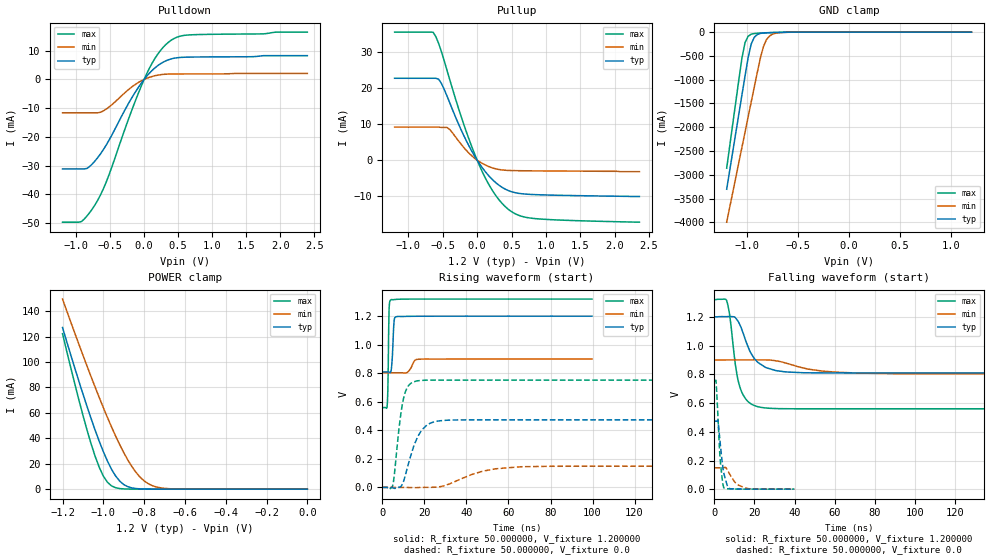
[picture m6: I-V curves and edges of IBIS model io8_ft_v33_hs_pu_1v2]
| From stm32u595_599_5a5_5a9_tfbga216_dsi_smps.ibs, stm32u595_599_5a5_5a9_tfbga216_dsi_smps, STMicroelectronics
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|   Model io8_ft_v33_hs_pu_1v2
[Model]  io8_ft_v33_hs_pu_1v2
Model_type I/O
Polarity   Non-Inverting
Enable   Active-Low
Vinl =   0.360000V
Vinh =   0.840000V
Vmeas =  0.600000V
Cref =   50.000000pF
Rref =   100.000000M
Vref =   0.0V
C_comp   2.887200pF   2.816900pF   2.935200pF
[Temperature Range]   25.000000   0.140000k   -40.000000
[Pullup Reference]   1.200000V   0.900000V   1.320000V
[Pulldown Reference]   0.0V   0.0V   0.0V
[POWER Clamp Reference]   1.200000V   0.900000V   1.320000V
[GND Clamp Reference]   0.0V   0.0V   0.0V
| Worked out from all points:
|   slope of the pulldown table from 0 to 0.18 V, typ, clamps not added: 40.7 ohm
|   slope of the pullup table from 0 to 0.18 V, typ, clamps not added: 39.5 ohm
|   GND clamp passes 1 mA (typ) near -0.51 V on its own axis
|   POWER clamp passes 1 mA (typ) near -0.86 V on its own axis
|   rising waveform, R_fixture 50.000000, V_fixture 1.200000: 20-80 % time 756ps typ, 2.05ns min, 445ps max; typ from 0.809 V to 1.2 V
|   rising waveform, R_fixture 50.000000, V_fixture 0.0: 20-80 % time 6.66ns typ, 16.9ns min, 3.63ns max; typ from 0.001 V to 0.474 V
|   falling waveform, R_fixture 50.000000, V_fixture 1.200000: 20-80 % time 7.98ns typ, 18.6ns min, 4.69ns max; typ from 1.2 V to 0.809 V
|   falling waveform, R_fixture 50.000000, V_fixture 0.0: 20-80 % time 2.51ns typ, 4.77ns min, 1.85ns max; typ from 0.474 V to 0.001 V
[Pulldown]
|Voltage   I(typ)   I(min)   I(max)
-1.2V     -31.16mA   -11.61mA   -49.71mA
-920mV    -31.16mA   -11.61mA   -49.49mA
-840mV    -31mA      -11.61mA   -47.54mA
-720mV    -28.32mA   -11.61mA   -43.58mA
-560mV    -22.95mA   -10.37mA   -35.89mA
-200mV    -7.146mA   -2.964mA   -11.89mA
0V        0A         0A         0A
160mV     4.047mA    1.298mA    7.361mA
360mV     6.869mA    1.87mA     13mA
480mV     7.543mA    1.91mA     14.69mA
640mV     7.765mA    1.923mA    15.46mA
2.4V      8.292mA    2.092mA    16.49mA
[Pullup]
|Voltage   I(typ)   I(min)   I(max)
-1.2V     22.73mA    9.162mA    35.55mA
-640mV    22.73mA    9.162mA    35.51mA
-560mV    22.48mA    9.162mA    32.41mA
-520mV    21.33mA    9.091mA    30.16mA
-400mV    15.99mA    8.534mA    22.45mA
-200mV    7.069mA    3.642mA    10.26mA
40mV      -1.16mA    -508.1uA   -1.774mA
240mV     -5.73mA    -2.256mA   -8.953mA
480mV     -8.639mA   -2.877mA   -14.04mA
640mV     -9.31mA    -2.942mA   -15.55mA
880mV     -9.601mA   -2.986mA   -16.29mA
2.36V     -10.1mA    -3.2mA     -17.23mA
[GND_clamp]
|Voltage   I(typ)   I(min)   I(max)
-1.2V     -3.305A    -3.998A    -2.862A
-1.05V    -1.316A    -2.418A    -539.3mA
-1.02V    -921mA     -2.103A    -218.8mA
-990mV    -539.5mA   -1.788A    -87.43mA
-960mV    -252.1mA   -1.474A    -44.36mA
-930mV    -110.5mA   -1.16A     -30.32mA
-870mV    -28.03mA   -549.1mA   -21.09mA
-840mV    -18.43mA   -305.6mA   -18.27mA
-810mV    -13.9mA    -159.7mA   -15.73mA
-780mV    -11.23mA   -82.35mA   -13.37mA
-600mV    -2.976mA   -4.272mA   -3.058mA
1.2V      0A         14.74nA    0A
[POWER_clamp]
|Voltage   I(typ)   I(min)   I(max)
-1.2V     127mA      149.4mA    122.2mA
-1.12V    84.98mA    114mA      70.29mA
-1.06V    55.52mA    88.42mA    35.69mA
-1.02V    37.64mA    72.04mA    17.19mA
-1V       29.52mA    64.13mA    10.33mA
-960mV    15.7mA     48.99mA    2.597mA
-900mV    3.636mA    28.77mA    209uA
-840mV    503.6uA    13.24mA    43.76uA
-800mV    129.7uA    6.535mA    43.76uA
-740mV    27.38uA    1.727mA    43.76uA
-620mV    25.25uA    82.57uA    35.67uA
0V        0A         17.33nA    0A
[Ramp]
| variable   typ   min   max
dV/dt_r  0.28389/6.64763n   89.03386m/16.87712n 0.45097/3.62302n
dV/dt_f  0.23431/7.97402n   57.82800m/18.56443n 0.45609/4.67810n
R_load = 50.000000
[Rising Waveform]
R_fixture= 50.000000
V_fixture= 1.200000
V_fixture_min= 0.900000
V_fixture_max= 1.320000
|time   V(typ)   V(min)   V(max)
0s        809.5mV    803.6mV    559.9mV
2.402ns   809.6mV    803.6mV    593.6mV
2.603ns   809.5mV    803.6mV    678.5mV
3.203ns   808.1mV    803.6mV    1.254V
4.204ns   822.5mV    803.6mV    1.316V
5.606ns   1.168V     803.6mV    1.316V
6.607ns   1.196V     803.6mV    1.318V
11.81ns   1.199V     805.9mV    1.32V
17.02ns   1.2V       898.1mV    1.32V
99.7ns    1.2V       900mV      1.32V
[Rising Waveform]
R_fixture= 50.000000
V_fixture= 0.0
V_fixture_min= 0.0
V_fixture_max= 0.0
|time   V(typ)   V(min)   V(max)
0s        599uV      600uV      555.1uV
4.805ns   -2.048mV   601.4uV    8.21mV
8.008ns   1.126mV    606.7uV    424.7mV
10.01ns   40.29mV    645.7uV    619.3mV
12.41ns   166.4mV    -255.2uV   712.8mV
16.42ns   342.9mV    -1.167mV   746.4mV
21.22ns   438mV      880.5uV    751.7mV
30.43ns   470.8mV    16.97mV    752mV
65.67ns   473.7mV    145mV      752.1mV
199.4ns   473.8mV    149mV      752.1mV
[Falling Waveform]
R_fixture= 50.000000
V_fixture= 1.200000
V_fixture_min= 0.900000
V_fixture_max= 1.320000
|time   V(typ)   V(min)   V(max)
0s        1.2V       900mV      1.32V
6.006ns   1.201V     900.3mV    1.316V
7.608ns   1.202V     900.6mV    1.213V
10.41ns   1.195V     900.7mV    871.1mV
12.41ns   1.153V     900.5mV    725.4mV
16.02ns   1.019V     900.5mV    621.5mV
21.62ns   884mV      900.5mV    574.9mV
35.64ns   816.6mV    878.4mV    560.5mV
72.07ns   809.5mV    808.4mV    559.9mV
199.4ns   809.5mV    803.6mV    559.9mV
[Falling Waveform]
R_fixture= 50.000000
V_fixture= 0.0
V_fixture_min= 0.0
V_fixture_max= 0.0
|time   V(typ)   V(min)   V(max)
0s        473.8mV    149mV      752.1mV
800.8ps   473.5mV    149mV      749.2mV
1.762ns   472.3mV    149mV      502.7mV
2.963ns   308.8mV    149mV      190.7mV
4.164ns   157mV      148.9mV    40.48mV
4.885ns   100.4mV    150.7mV    7.664mV
7.207ns   7.092mV    115mV      2.757mV
10.89ns   2.37mV     39.87mV    1.064mV
15.3ns    1.218mV    9.697mV    713.3uV
39.88ns   599uV      600uV      555.1uV
